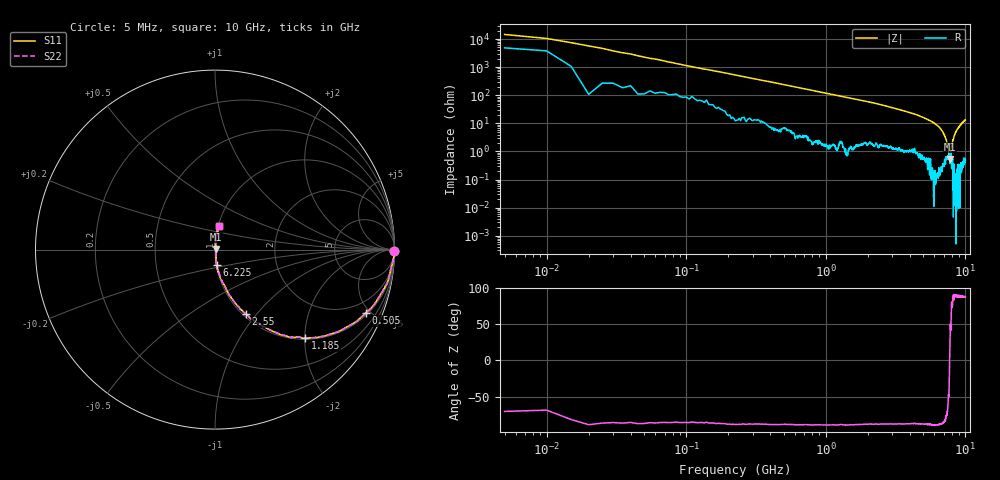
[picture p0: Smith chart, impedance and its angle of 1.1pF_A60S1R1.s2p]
! Amotech Co.,Ltd.
! http://www.amotech.co.kr/
! Part Number: A60S1R1
! These Parameters are Measured in Series Mode Connection
! Operation Temp=25[degC], DC Bias Voltage=0[V]
! Freq. Start=5[MHz] Stop=10[GHz], 2000[Steps]
! Date: Monday, July 13, 2020, 01:48:33
# GHZ S RI R 50.000000
!Freq.(Hz) S11(Real) S11(Imag) S21(Real) S21(Imag) S12(Real) S12(Imag) S22(Real) S22(Imag)
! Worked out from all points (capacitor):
!   2000 points, 5 MHz to 10 GHz, reference 50 ohm
!   read as one part in series: C = 1.39 pF near 55 MHz
!   lowest |Z| = 540 mohm at 7.79 GHz (marker M1)
!   series resonance near 7.709 GHz, so ESL is about 310 pH
!   S11 on the Smith chart (normalised r, x): 5 MHz: open; 505 MHz: 1.13, -4.72; 1.185 GHz: 1.02, -2.01; 2.55 GHz: 1.03, -0.88; 6.225 GHz: 1.00, -0.18; 10 GHz: 1.01, +0.27
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0.005  0.9977 -0.00646  0.00233 0.00646  0.00233 0.00646  0.9977 -0.00646
0.075  0.9913 -0.0648  0.00868 0.0648  0.00868 0.0648  0.9913 -0.0648
0.145  0.9777 -0.1212  0.0223 0.1212  0.0223 0.1212  0.9777 -0.1212
0.295  0.9347 -0.2315  0.0653 0.2315  0.0653 0.2315  0.9347 -0.2315
0.505  0.841 -0.3523  0.159 0.3523  0.159 0.3523  0.841 -0.3523
1.185  0.5023 -0.4941  0.4977 0.4941  0.4977 0.4941  0.5023 -0.4941
1.675  0.338 -0.4615  0.662 0.4615  0.662 0.4615  0.338 -0.4615
2.55  0.1727 -0.3602  0.8273 0.3602  0.8273 0.3602  0.1727 -0.3602
3.34  0.0979 -0.2763  0.9021 0.2763  0.9021 0.2763  0.0979 -0.2763
5.005  0.0305 -0.1545  0.9695 0.1545  0.9695 0.1545  0.0305 -0.1545
6.225  0.00897 -0.0869  0.991 0.0869  0.991 0.0869  0.00897 -0.0869
6.67  0.00642 -0.0621  0.9936 0.0621  0.9936 0.0621  0.00642 -0.0621
7.25  0.00636 -0.0269  0.9936 0.0269  0.9936 0.0269  0.00636 -0.0269
7.46  0.00644 -0.0155  0.9936 0.0155  0.9936 0.0155  0.00644 -0.0155
7.625  0.00543 -0.00621  0.9946 0.00621  0.9946 0.00621  0.00543 -0.00621
7.79  0.00379 0.00382  0.9962 -0.00382  0.9962 -0.00382  0.00379 0.00382
7.925  0.00583 0.0132  0.9942 -0.0132  0.9942 -0.0132  0.00583 0.0132
8.02  0.00398 0.0144  0.996 -0.0144  0.996 -0.0144  0.00398 0.0144
8.115  0.00453 0.0247  0.9955 -0.0247  0.9955 -0.0247  0.00453 0.0247
8.335  0.00126 0.0375  0.9987 -0.0375  0.9987 -0.0375  0.00126 0.0375
8.94  0.00612 0.0712  0.9939 -0.0712  0.9939 -0.0712  0.00612 0.0712
10  0.0221 0.1298  0.9779 -0.1298  0.9779 -0.1298  0.0221 0.1298
